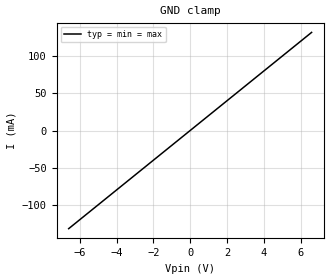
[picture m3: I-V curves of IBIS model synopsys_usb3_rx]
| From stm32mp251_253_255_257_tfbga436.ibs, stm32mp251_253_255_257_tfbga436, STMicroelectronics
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[Model] synopsys_usb3_rx
Model_type Input
C_comp 657.212f 509.522f 695.934f
Vinl = 0.49
Vinh = 0.51
[Temperature_Range] 25 125 0
[Voltage Range] 1.0 1.0 1.0
[Algorithmic Model]
Executable Linux_GCC_64 synopsys_usb3_rx_ami_x64.so synopsys_usb3_rx_ami.ami
Executable Windows_cl_64 synopsys_usb3_rx_ami_x64.dll synopsys_usb3_rx_ami.ami
Executable Windows_cl_32 synopsys_usb3_rx_ami.dll synopsys_usb3_rx_ami.ami
[End Algorithmic Model]
[GND Clamp]
-6.6V     -132mA     -132mA     -132mA
0V        0A         0A         0A
6.6V      132mA      132mA      132mA
[Power Clamp]
-6.6V     0A         0A         0A
0V        0A         0A         0A
6.6V      0A         0A         0A
